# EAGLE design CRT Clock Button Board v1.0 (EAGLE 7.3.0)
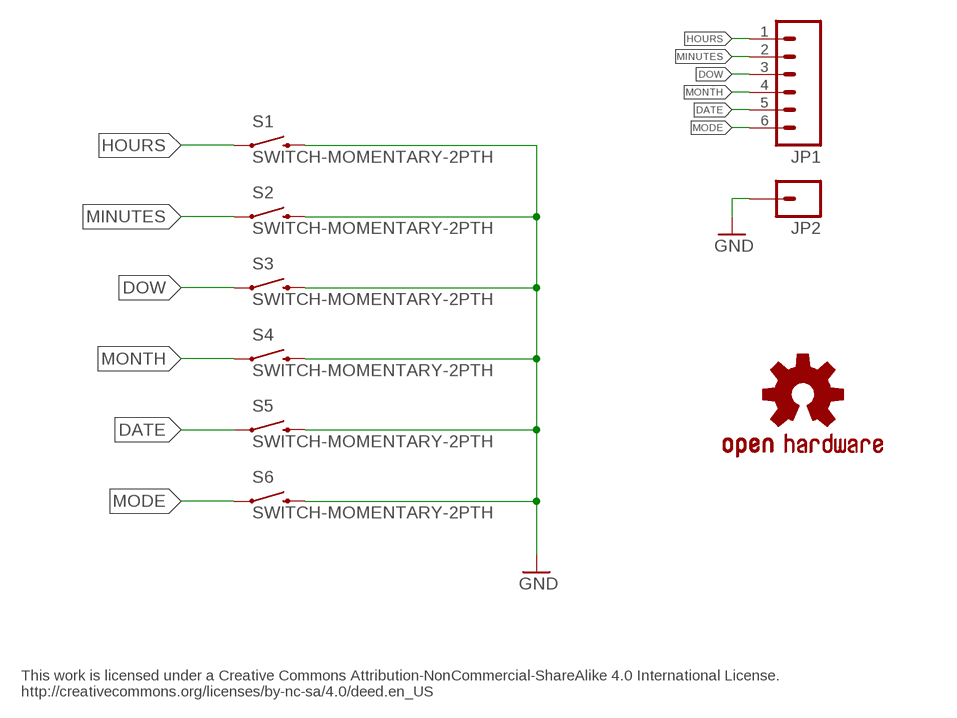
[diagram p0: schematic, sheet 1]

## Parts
JP1  M06NO_SILK_FEMALE_PTH  [1X06_NO_SILK]
JP2  M01NOSILK-KIT  [1X01NS-KIT]
S1  SWITCH-MOMENTARY-2PTH  [TACTILE-PTH]
S2  SWITCH-MOMENTARY-2PTH  [TACTILE-PTH]
S3  SWITCH-MOMENTARY-2PTH  [TACTILE-PTH]
S4  SWITCH-MOMENTARY-2PTH  [TACTILE-PTH]
S5  SWITCH-MOMENTARY-2PTH  [TACTILE-PTH]
S6  SWITCH-MOMENTARY-2PTH  [TACTILE-PTH]
U$7  OSHW-LOGOS  [OSHW-LOGO-S]

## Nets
DATE: JP1.5 S5.1
DOW: JP1.3 S3.1
GND: JP2.1 S1.3 S2.3 S3.3 S4.3 S5.3 S6.3
HOURS: JP1.1 S1.1
MINUTES: JP1.2 S2.1
MODE: JP1.6 S6.1
MONTH: JP1.4 S4.1

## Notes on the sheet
- This work is licensed under a Creative Commons Attribution-NonCommercial-ShareAlike 4.0 International License.
  http://creativecommons.org/licenses/by-nc-sa/4.0/deed.en_US

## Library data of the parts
JP1 = SparkFun-Connectors:M06: Header 6 Standard 6-pin 0.1" header. Use with straight break away headers (SKU : PRT-00116), right angle break away headers (PRT-00553), swiss pins (PRT-00743), machine pins (PRT-00117), and female headers (PRT-00115). Molex polarized connector foot print use with SKU : PRT-08094 with associated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; PROD_ID: CONN-08437
JP2 = SparkFun-Connectors:M01: Header 1
S1-S6 = SparkFun:SWITCH-MOMENTARY-2
U$7 = SparkFun:OSHW-LOGO: Open Source Hardware Logo This logo indicates the piece of hardware it is found on incorporates a OSHW license and/or adheres to the definition of open source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

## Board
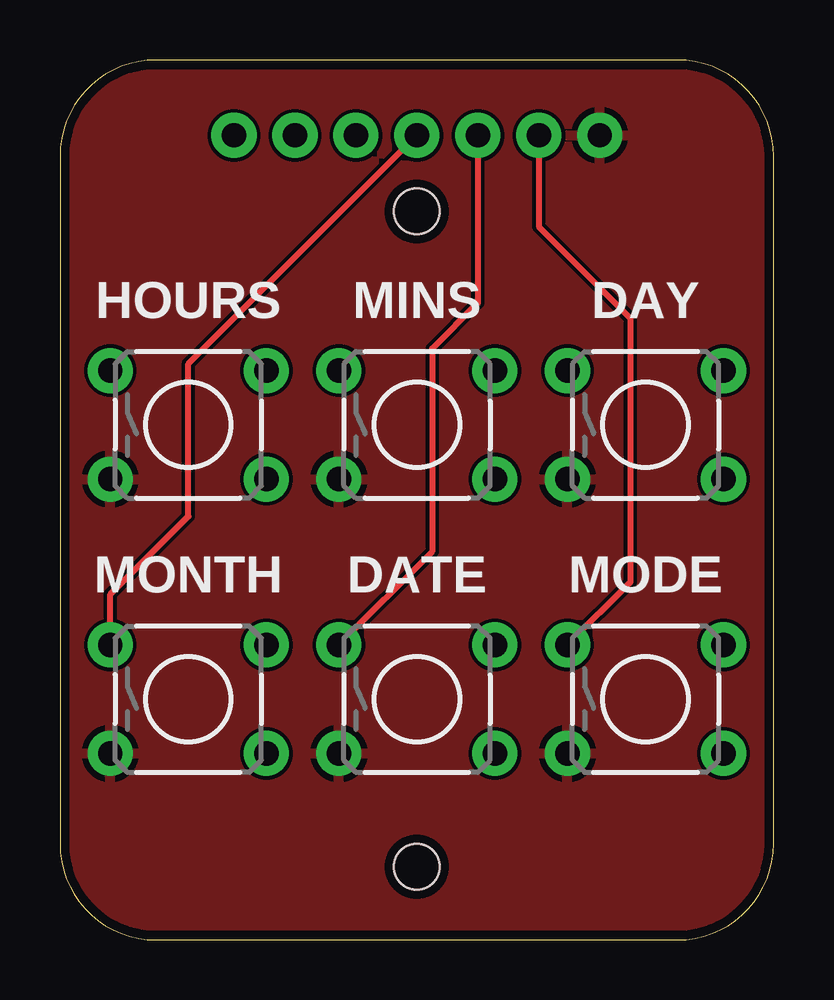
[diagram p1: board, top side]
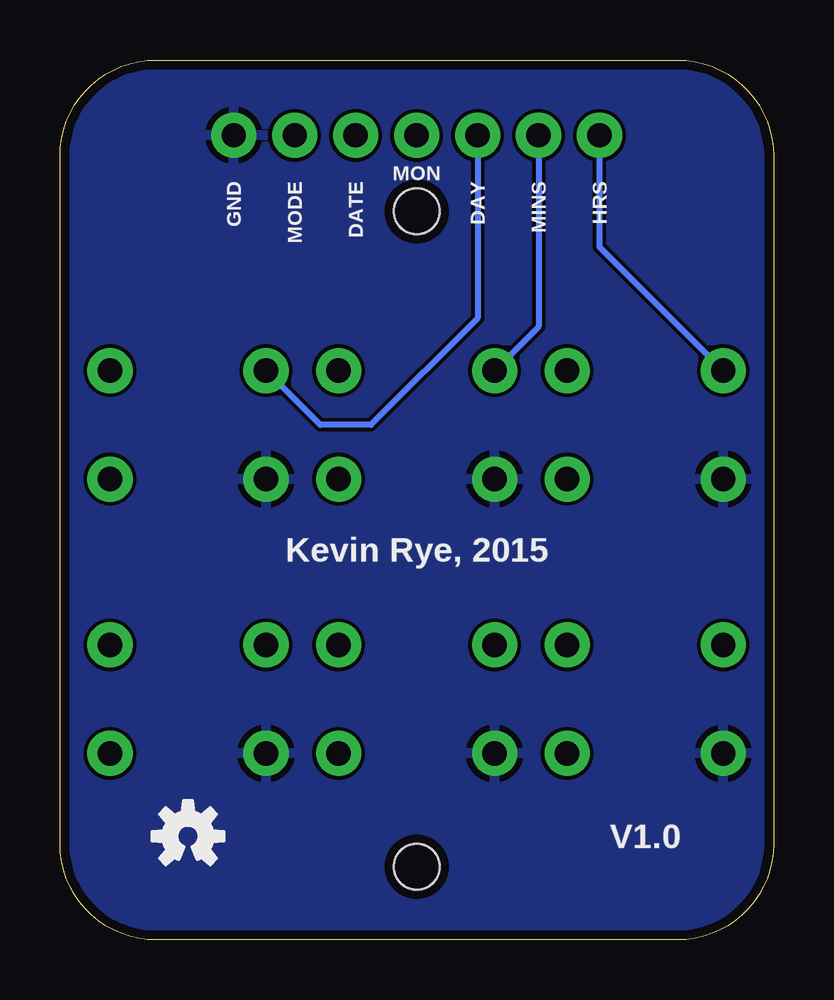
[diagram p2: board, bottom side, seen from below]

Size 29.73 x 36.66 mm. Coordinates in mm from the lower left corner, seen from the top.
Copper layers (1*16): Top 0.0356mm / dielectric 1.5011mm / Bottom 0.0356mm
Design rules "LaenPCBOrder": minimum track width 6mil, minimum drill 13mil, track to track 6mil, track to pad 6mil, pad to pad 6mil, via to via 6mil, smd to smd 6mil, copper to edge 15mil, drill to drill 6mil, minimum pad ring 7mil, minimum via ring 7mil, stop-mask expansion 3mil, vias tented up to drill 0mil, thermal gap 10mil
Holes 1.9 mm at 14.87,3.05 14.87,30.35

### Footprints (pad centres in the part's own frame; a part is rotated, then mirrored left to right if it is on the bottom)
1X06_NO_SILK = drill 1.016 pad 1.88: 1 0,0; 2 2.54,0; 3 5.08,0; 4 7.62,0; 5 10.16,0; 6 12.7,0
1X01NS-KIT = drill 1.016 pad 1.88: 1 0,0
TACTILE-PTH = drill 1.016 pad 1.88: 1 -3.251,2.261; 2 3.251,2.261; 3 -3.251,-2.261; 4 3.251,-2.261

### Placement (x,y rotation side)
JP1  7.25,33.53 0 top
JP2  22.49,33.53 0 top
S1  5.35,21.46 0 top
S2  14.87,21.46 0 top
S3  24.4,21.46 0 top
S4  5.35,10.03 0 top
S5  14.87,10.03 0 top
S6  24.4,10.03 0 top
U$2  [DP50XX_BUTTONBREAKOUT2]  0.52,0 0 top
U$7  24.4,4.32 0 bottom

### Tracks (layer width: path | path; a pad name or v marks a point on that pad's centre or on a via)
DATE
  Top 0.254: JP1.5 17.41,26.54 15.51,24.64 15.51,16.18 S5.1
DOW
  Bottom 0.254: JP1.3 12.33,25.91 16.78,21.46 18.88,21.46 S3.1
GND
  pour Top: -1,37.97 30.75,37.97 30.75,-1.4 -1,-1.4
  pour Bottom: -0.37,37.34 30.11,37.34 30.11,-0.76 -0.37,-0.76
HOURS
  Bottom 0.254: JP1.1 7.25,28.88 S1.1
MINUTES
  Bottom 0.254: JP1.2 9.79,25.55 S2.1
MODE
  Top 0.254: JP1.6 19.95,29.72 23.76,25.91 23.76,14.91 S6.1
MONTH
  Top 0.254: S4.1 2.09,14.4 5.35,17.65 5.35,24 JP1.4

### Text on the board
Unrouted: This work is licensed under a Creative Commons Attribution-NonCommercial-ShareAlike 4.0 International License. / http://creativecommons.org/licenses/by-nc-sa/4.0/deed.en_US
tNames: HOURS | MINS | DAY | MONTH | DATE | MODE
bNames: HRS | MINS | DAY | MON | DATE | MODE | GND | Kevin Rye, 2015 | V1.0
